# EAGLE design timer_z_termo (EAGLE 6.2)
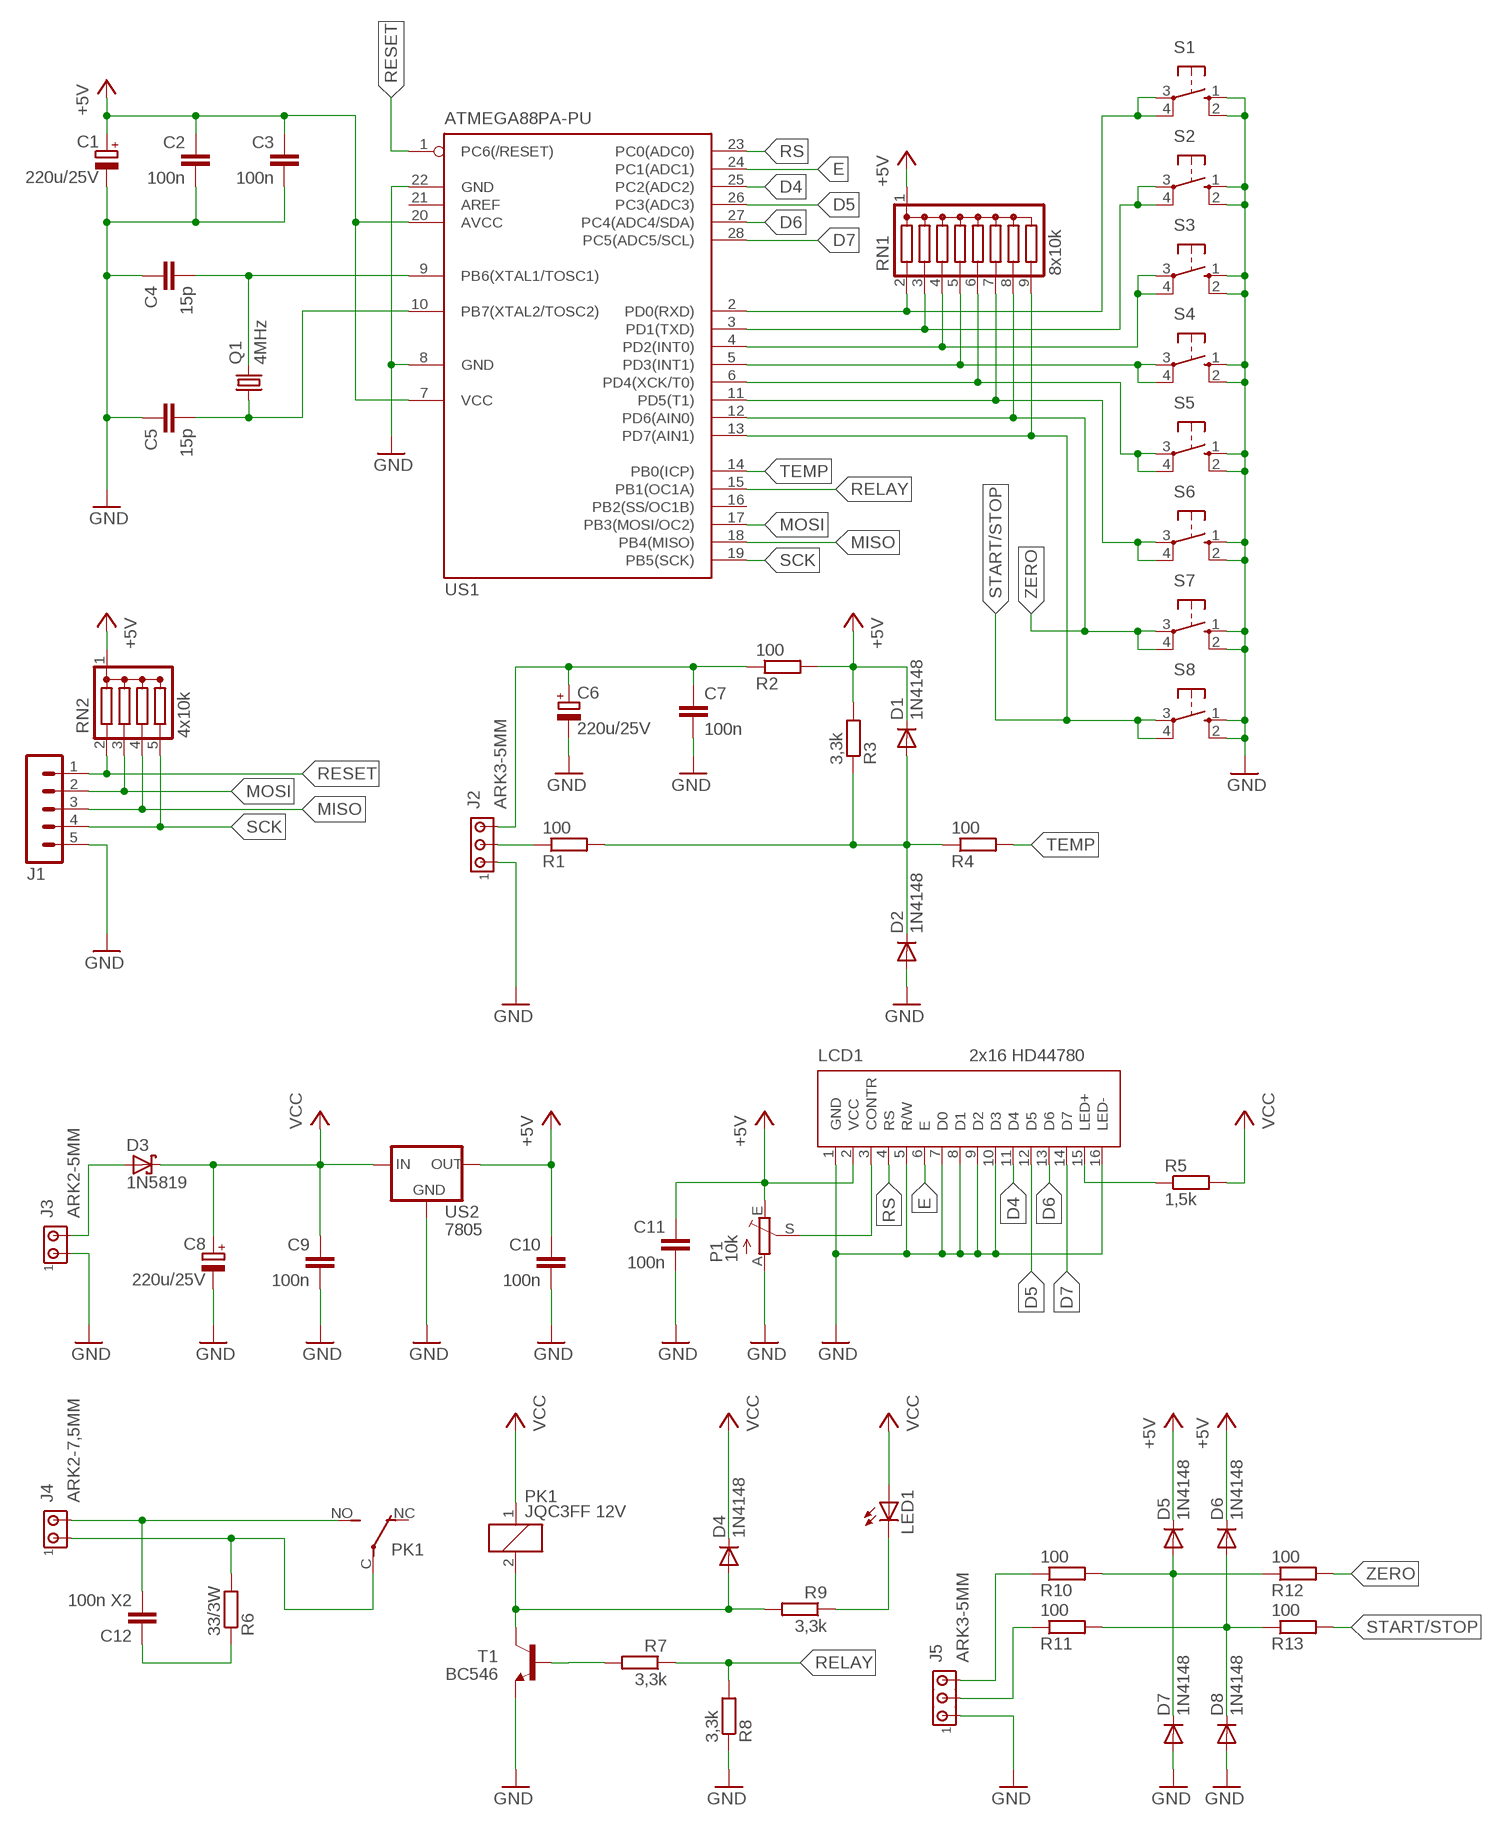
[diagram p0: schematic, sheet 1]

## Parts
C1  220u/25V  CPOL-EUE2.5-7  [E2,5-7]
C2  100n  C-EU050-025X075  [C050-025X075]
C3  100n  C-EU050-025X075  [C050-025X075]
C4  15p  C-EU050-025X075  [C050-025X075]
C5  15p  C-EU050-025X075  [C050-025X075]
C6  220u/25V  CPOL-EUE2.5-7  [E2,5-7]
C7  100n  C-EU050-025X075  [C050-025X075]
C8  220u/25V  CPOL-EUE2.5-7  [E2,5-7]
C9  100n  C-EU050-025X075  [C050-025X075]
C10  100n  C-EU050-025X075  [C050-025X075]
C11  100n  C-EU050-025X075  [C050-025X075]
C12  100n X2  C-EU102_152-062X184  [C102_152-062X184]
D1  1N4148  BAT81  [DO34-7]
D2  1N4148  BAT81  [DO34-7]
D3  1N5819  SCHOTTKY-DIODEF126Z12  [F126Z12]
D4  1N4148  BAT81  [DO34-7]
D5  1N4148  BAT81  [DO34-7]
D6  1N4148  BAT81  [DO34-7]
D7  1N4148  BAT81  [DO34-7]
D8  1N4148  BAT81  [DO34-7]
J1  MA05-1  [MA05-1]
J2  ARK3-5MM  [3PIN-5MM]
J3  ARK2-5MM  [2PIN-5MM]
J4  ARK2-7,5MM  [2PIN-7,5MM]
J5  ARK3-5MM  [3PIN-5MM]
LCD1  2x16 HD44780  LCD_2X16-NAD-ELEMENTAMI  [LCD_HD44780_2X16_NAD-ELEMENTAMI]
LED1  LED5MM  [LED5MM]
P1  10k  TRIM_EU-CA6V  [CA6V]
PK1  JQC3FF 12V  PK_POJED-JQC-3FG  [PK_POJED_JQC-3FG]
Q1  4MHz  CRYSTALHC49U-V  [HC49U-V]
R1  100  R-EU_0207/7  [0207/7]
R2  100  R-EU_0207/7  [0207/7]
R3  3,3k  R-EU_0207/7  [0207/7]
R4  100  R-EU_0207/7  [0207/7]
R5  1,5k  R-EU_0207/7  [0207/7]
R6  33/3W  R-EU_0617/17  [0617/17]
R7  3,3k  R-EU_0207/7  [0207/7]
R8  3,3k  R-EU_0207/7  [0207/7]
R9  3,3k  R-EU_0207/7  [0207/7]
R10  100  R-EU_0207/7  [0207/7]
R11  100  R-EU_0207/7  [0207/7]
R12  100  R-EU_0207/7  [0207/7]
R13  100  R-EU_0207/7  [0207/7]
RN1  8x10k  DRAB_REZ_1X8-SIL9  [RN-9]
RN2  4x10k  DRAB_REZ_1X4  [RN-5]
S1  10-XX  [B3F-10XX]
S2  10-XX  [B3F-10XX]
S3  10-XX  [B3F-10XX]
S4  10-XX  [B3F-10XX]
S5  10-XX  [B3F-10XX]
S6  10-XX  [B3F-10XX]
S7  10-XX  [B3F-10XX]
S8  10-XX  [B3F-10XX]
T1  BC546  BC546A  [TO92-EBC]
US1  ATMEGA88PA-PU  MEGA8-P  [DIL28-3]
US2  7805  78XXL  [78XXL]

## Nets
+5V: C1.+ C2.1 C3.1 C10.1 C11.1 D1.C D5.C D6.C LCD1.2(VCC) P1.E R2.2 R3.2 RN1.1(C) RN2.1(C) US1.7(VCC) US1.20(AVCC) US2.OUT
D4: LCD1.11(D4) US1.25(PC2(ADC2))
D5: LCD1.12(D5) US1.26(PC3(ADC3))
D6: LCD1.13(D6) US1.27(PC4(ADC4/SDA))
D7: LCD1.14(D7) US1.28(PC5(ADC5/SCL))
E: LCD1.6(E) US1.24(PC1(ADC1))
GND: C1.- C2.2 C3.2 C4.1 C5.1 C6.- C7.2 C8.- C9.2 C10.2 C11.2 D2.A D7.A D8.A J1.5 J2.P$1 J3.P$1 J5.P$1 LCD1.1(GND) LCD1.5(R/W) LCD1.7(D0) LCD1.8(D1) LCD1.9(D2) LCD1.10(D3) LCD1.16(LED-) P1.A R8.1 S1.1(S) S1.2(S1) S2.1(S) S2.2(S1) S3.1(S) S3.2(S1) S4.1(S) S4.2(S1) S5.1(S) S5.2(S1) S6.1(S) S6.2(S1) S7.1(S) S7.2(S1) S8.1(S) S8.2(S1) T1.E US1.8(GND) US1.22(GND) US2.GND
MISO: J1.3 RN2.4 US1.18(PB4(MISO))
MOSI: J1.2 RN2.3 US1.17(PB3(MOSI/OC2))
N$1: LCD1.3(CONTR) P1.S
N$2: C12.2 J4.P2 PK1.NO
N$3: C5.2 Q1.1 US1.10(PB7(XTAL2/TOSC2))
N$4: C4.2 Q1.2 US1.9(PB6(XTAL1/TOSC1))
N$5: RN1.2 S1.3(P) S1.4(P1) US1.2(PD0(RXD))
N$6: LCD1.15(LED+) R5.1
N$7: R7.2 T1.B
N$8: D3.A J3.P$2
N$9: D4.A PK1.2 R9.2 T1.C
N$10: RN1.3 S2.3(P) S2.4(P1) US1.3(PD1(TXD))
N$11: J4.P1 PK1.C(COM) R6.2
N$12: C12.1 R6.1
N$13: RN1.4 S3.3(P) S3.4(P1) US1.4(PD2(INT0))
N$14: RN1.5 S4.3(P) S4.4(P1) US1.5(PD3(INT1))
N$15: RN1.6 S5.3(P) S5.4(P1) US1.6(PD4(XCK/T0))
N$16: RN1.7 S6.3(P) S6.4(P1) US1.11(PD5(T1))
N$19: C6.+ C7.1 J2.P$3 R2.1
N$20: J2.P$2 R1.1
N$21: D1.A D2.C R1.2 R3.1 R4.1
N$22: LED1.K(C) R9.1
N$23: D5.A D7.C R10.2 R12.1
N$24: D6.A D8.C R11.2 R13.1
N$25: J5.P$2 R11.1
N$26: J5.P$3 R10.1
RELAY: R7.1 R8.2 US1.15(PB1(OC1A))
RESET: J1.1 RN2.2 US1.1(PC6(/RESET))
RS: LCD1.4(RS) US1.23(PC0(ADC0))
SCK: J1.4 RN2.5 US1.19(PB5(SCK))
START/STOP: R13.2 RN1.9 S8.3(P) S8.4(P1) US1.13(PD7(AIN1))
TEMP: R4.2 US1.14(PB0(ICP))
VCC: C8.+ C9.1 D3.C D4.C LED1.A PK1.1 R5.2 US2.IN
ZERO: R12.2 RN1.8 S7.3(P) S7.4(P1) US1.12(PD6(AIN0))
Unconnected: PK1.NC US1.16(PB2(SS/OC1B)) US1.21(AREF)

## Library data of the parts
C1 C6 C8 = rcl:CPOL-EU: POLARIZED CAPACITOR, European symbol
C2-C5 C7 C9-C12 = rcl:C-EU: CAPACITOR, European symbol
D1 D2 D4-D8 = diode:BAT81: DIODE
D3 = diode:SCHOTTKY-DIODE: Schottky Diode
J1 = zlacza_futrzak:MA05-1: PIN HEADER; OC_FARNELL: unknown; OC_NEWARK: unknown
J2 J5 = zlacza_futrzak:ARK3: ARK 3 Raster 5mm i 3,5mm
J3 J4 = zlacza_futrzak:ARK2: ARK 2
LCD1 = inne_futrzak:LCD_2X16
LED1 = led:LED: LED
P1 = pot:TRIM_EU-: POTENTIOMETER
PK1 = inne_futrzak:PK_POJED
Q1 = crystal:CRYSTAL: CRYSTAL; OC_FARNELL: 1666969; OC_NEWARK: unknown
R1-R13 = rcl:R-EU_: RESISTOR, European symbol
RN1 = inne_futrzak:DRAB_REZ_1X8
RN2 = inne_futrzak:DRAB_REZ_1X4
S1-S8 = switch-omron:10-XX: OMRON SWITCH; MPN: B3F-1000; OC_FARNELL: 176432; OC_NEWARK: 36M3542
T1 = transistor-npn:BC546*: NPN Transistor
US1 = atmel:MEGA8-P: MICROCONTROLLER 8 Kbytes FLASH, 1 kbytes SRAM, 512 bytes EEPROM, USART, 4-channel 10 bit ADC, 2-channel 8 bit ADC Pin compatible with Atmega48, ATMega88, ATMega168 Source: avr.lbr; OC_FARNELL: unknown; OC_NEWARK: unknown
US2 = v-reg:78XXL: VOLTAGE REGULATOR

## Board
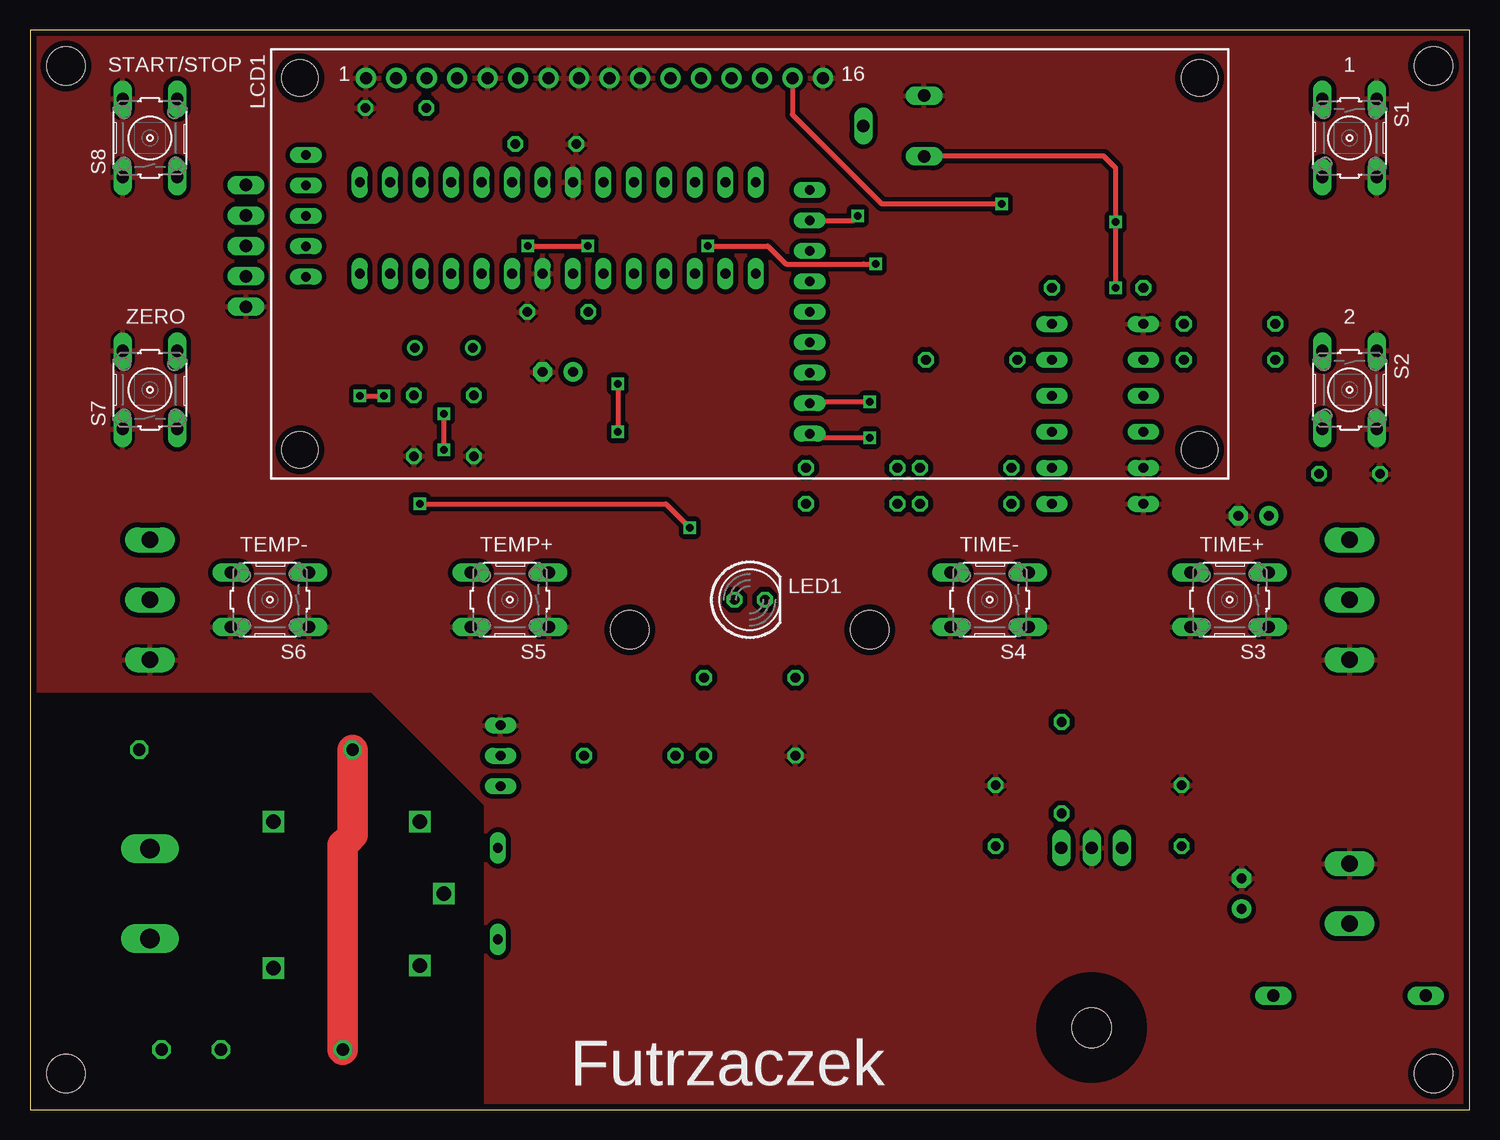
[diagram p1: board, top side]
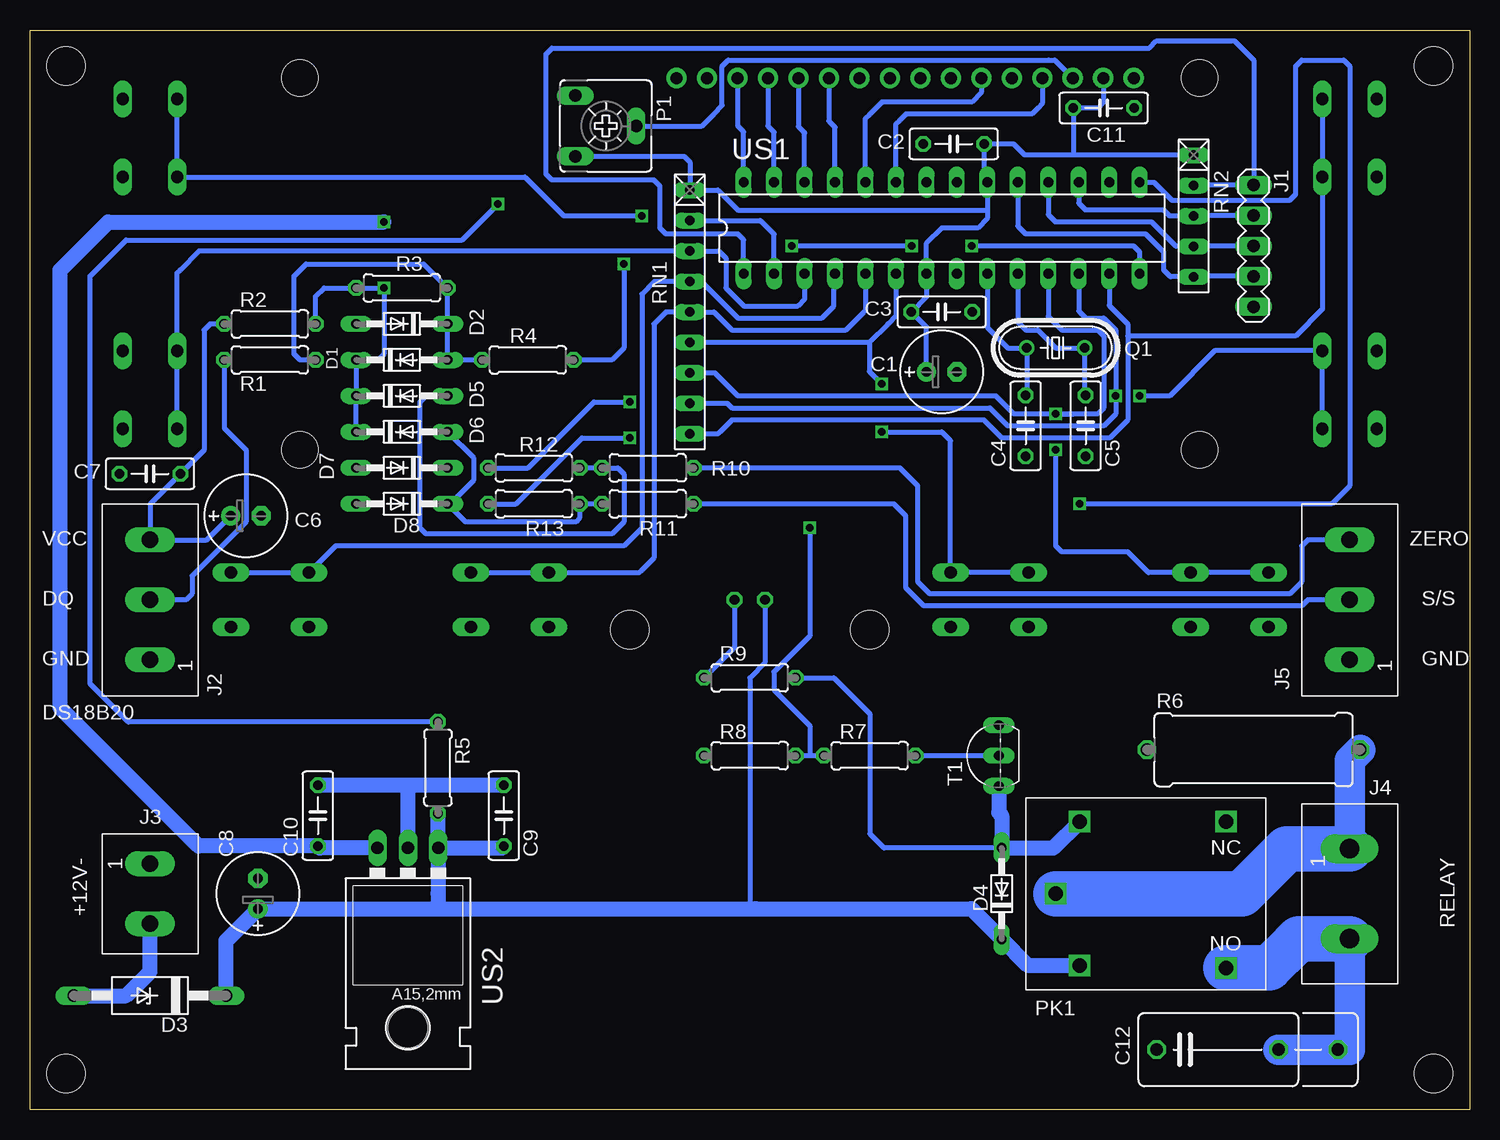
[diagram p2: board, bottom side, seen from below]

Size 120 x 90 mm. Coordinates in mm from the lower left corner, seen from the top.
Outline: 0,0 120,0 120,90 0,90 0,0
Copper layers (1*16): Top 0.035mm / dielectric 1.5mm / Bottom 0.035mm
Design rules: minimum track width 10mil, minimum drill 23mil, track to track 8mil, track to pad 8mil, pad to pad 8mil, via to via 8mil, smd to smd 8mil, copper to edge 20mil, drill to drill 8mil, minimum pad ring 10mil, minimum via ring 8mil, stop-mask expansion 4mil, vias tented up to drill 0mil, thermal gap 10mil
Holes 3.2 mm at 3,87 117,87 50,40 70,40 3,3 117,3

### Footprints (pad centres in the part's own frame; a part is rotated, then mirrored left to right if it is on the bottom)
E2,5-7 = drill 0.813 pad 1.6: + -1.27,0 | drill 0.813 pad 1.6 octagon: - 1.27,0
C050-025X075 = drill 0.813 octagon: 1 -2.54,0; 2 2.54,0
C102_152-062X184 = drill 1.016 octagon: 1 -5.08,0; 2 5.08,0; 3 10.033,0
DO34-7 = drill 0.813 long: A 3.81,0; C -3.81,0
F126Z12 = drill 1.016 long: A 6.35,0; C -6.35,0
MA05-1 = drill 1.016 long: 1 -5.08,0; 2 -2.54,0; 3 0,0; 4 2.54,0; 5 5.08,0
3PIN-5MM = drill 1.4 long: P$1 -5,0; P$2 0,0; P$3 5,0
2PIN-5MM = drill 1.4 long: P$1 -2.5,0; P$2 2.5,0
2PIN-7,5MM = drill 1.6 long: P1 -3.75,0; P2 3.75,0
LCD_HD44780_2X16_NAD-ELEMENTAMI = drill 1 pad 1.676: 1 -32,15.5; 2 -29.46,15.5; 3 -26.92,15.5; 4 -24.38,15.5; 5 -21.84,15.5; 6 -19.3,15.5; 7 -16.76,15.5; 8 -14.22,15.5; 9 -11.68,15.5; 10 -9.14,15.5; 11 -6.6,15.5; 12 -4.06,15.5; 13 -1.52,15.5; 14 1.02,15.5; 15 3.56,15.5; 16 6.1,15.5 | hole 3: -37.5,-15.5; 37.5,-15.5; -37.5,15.5; 37.5,15.5
LED5MM = drill 0.813 octagon: A -1.27,0; K 1.27,0
CA6V = drill 1.016 long: A -2.54,-2.54; E 2.54,-2.54; S 0,2.54
PK_POJED_JQC-3FG = drill 1.2 square: 1 5.5,6; 2 5.5,-6; C 7.5,0; NC -6.7,-6; NO -6.7,6.2
HC49U-V = drill 0.813: 1 -2.413,0; 2 2.413,0
0207/7 = drill 0.813 octagon: 1 -3.81,0; 2 3.81,0
0617/17 = drill 1.016 octagon: 1 -8.89,0; 2 8.89,0
RN-9 = drill 0.813 long: 1 -10.16,0; 2 -7.62,0; 3 -5.08,0; 4 -2.54,0; 5 0,0; 6 2.54,0; 7 5.08,0; 8 7.62,0; 9 10.16,0
RN-5 = drill 0.813 long: 1 -5.08,0; 2 -2.54,0; 3 0,0; 4 2.54,0; 5 5.08,0
B3F-10XX = drill 1.016 long: 1 -3.251,2.261; 2 3.251,2.261; 3 -3.251,-2.261; 4 3.251,-2.261
TO92-EBC = drill 0.813 long: B 0,-1.27; C -2.54,-1.27; E 2.54,-1.27
DIL28-3 = drill 0.813 long: 1 -16.51,-3.81; 2 -13.97,-3.81; 3 -11.43,-3.81; 4 -8.89,-3.81; 5 -6.35,-3.81; 6 -3.81,-3.81; 7 -1.27,-3.81; 8 1.27,-3.81; 9 3.81,-3.81; 10 6.35,-3.81; 11 8.89,-3.81; 12 11.43,-3.81; 13 13.97,-3.81; 14 16.51,-3.81; 15 16.51,3.81; 16 13.97,3.81; 17 11.43,3.81; 18 8.89,3.81; 19 6.35,3.81; 20 3.81,3.81; 21 1.27,3.81; 22 -1.27,3.81; 23 -3.81,3.81; 24 -6.35,3.81; 25 -8.89,3.81; 26 -11.43,3.81; 27 -13.97,3.81; 28 -16.51,3.81
78XXL = drill 1.016 long: GND 0,-3.81; IN -2.54,-3.81; OUT 2.54,-3.81 | hole 3.302: 0,11.176

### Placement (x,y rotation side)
C1  44,61.5 0 bottom
C2  43,80.5 180 bottom
C3  44,66.5 0 bottom
C4  37,57 90 bottom
C5  32,57 90 bottom
C6  102,49.5 0 bottom
C7  110,53 180 bottom
C8  101,18 90 bottom
C9  80.5,24.5 90 bottom
C10  96,24.5 90 bottom
C11  30.5,83.5 0 bottom
C12  21,5 0 bottom
D1  89,62.5 0 bottom
D2  89,65.5 180 bottom
D3  110,9.5 180 bottom
D4  39,18 90 bottom
D5  89,59.5 0 bottom
D6  89,56.5 0 bottom
D7  89,53.5 180 bottom
D8  89,50.5 180 bottom
J1  18,72 270 bottom
J2  110,42.5 90 bottom
J3  110,18 270 bottom
J4  10,18 270 bottom
J5  10,42.5 90 bottom
LCD1  60,70.5 0 top
LED1  60,42.5 0 top
P1  72,82 270 bottom
PK1  27,18 180 bottom
Q1  34.5,63.5 180 bottom
R1  100,62.5 0 bottom
R2  100,65.5 0 bottom
R3  89,68.5 180 bottom
R4  78.5,62.5 0 bottom
R5  86,28.5 270 bottom
R6  18,30 0 bottom
R7  50,29.5 0 bottom
R8  60,29.5 0 bottom
R9  60,36 0 bottom
R10  68.5,53.5 180 bottom
R11  68.5,50.5 180 bottom
R12  78,53.5 180 bottom
R13  78,50.5 180 bottom
RN1  65,66.5 270 bottom
RN2  23,74.5 270 bottom
S1  110,81 270 top
S2  110,60 270 top
S3  100,42.5 180 top
S4  80,42.5 180 top
S5  40,42.5 180 top
S6  20,42.5 180 top
S7  10,60 90 top
S8  10,81 90 top
T1  40.5,29.5 90 bottom
US1  44,73.5 0 bottom
US2  88.5,18 180 bottom

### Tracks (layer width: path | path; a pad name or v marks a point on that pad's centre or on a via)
+5V  (via drill 0.6)
  Top 0.406: v90.5,68.5 v90.5,74 90.5,78.5 89.5,79.5 74.58,79.5 P1.E
  Bottom 0.406: 40.19,75 US1.20 40.46,77.58 C2.1 38,80.5 37.08,79.58 33,79.58 | 40.19,75 40.19,74.31 41,73.5 44,73.5 45.27,72.23 US1.7 45.27,67.77 C3.1 45.27,65.23 C1.+ | RN2.1 33,79.58 | 33,79.58 33.04,79.62 C11.1 31,83.5 30.54,83.96 LCD1.2 | 40.19,75 61,75 62.66,76.66 RN1.1 65,79 65.46,79.46 P1.E | D6.C D5.C D1.C 91,62.5 90.5,63 v90.5,68.5 R3.2 95.5,68.5 96.19,67.81 R2.2
  Bottom 1.27: US2.OUT 95.85,21.81 C10.1 105.96,21.96 117.5,33.5 117.5,70 113.5,74 v90.5,74
D4
  Bottom 0.406: US1.25 52.89,81.89 53,82 53.4,82.4 LCD1.11
D5
  Bottom 0.406: US1.26 55.43,81.43 55.94,81.94 LCD1.12
D6
  Bottom 0.406: US1.27 57.97,81.47 58.48,81.98 LCD1.13
D7
  Bottom 0.406: US1.28 60.51,81.51 61,82 61.02,82.02 LCD1.14
E
  Bottom 0.406: LCD1.6 40.7,84.8 41.5,84 49,84 50,83 50.35,82.65 US1.24
GND
  Bottom 1.27: C9.2 88.5,27.04 | 88.5,27.04 C10.2 | US2.GND 88.5,27.04
  pour Top (isolate 0.406): 0,35 28.5,35 38,25.5 38,0 120,0 120,90 0,90
MISO
  Bottom 0.406: J1.3 22.96,72 RN2.4 24.46,71.96 26.5,74 34.5,74 35.11,74.61 US1.18
MOSI
  Bottom 0.406: J1.2 22.96,74.54 RN2.3 25,74.5 25.5,75 32,75 32.57,75.57 US1.17
N$1
  Bottom 0.406: P1.S 64,82 63,83 62.3,83.7 62.3,87 61.8,87.5 35.08,87.5 34.58,87.5 LCD1.3
N$2
  Bottom 2.54: J4.P2 10,5 C12.2
  Bottom 3.81: PK1.NO 16.7,11.8 14.75,13.75 | 14.75,13.75 14.5,14 | J4.P2 14.25,14.25 14.75,13.75
N$3
  Bottom 0.406: US1.10 37.65,65.65 37,65 36,65 34.5,63.5 Q1.1 32.09,59.63 C5.2
N$4
  Bottom 0.406: US1.9 40.19,65.19 38.5,63.5 Q1.2 36.91,59.63 C4.2
N$5  (via drill 0.6)
  Top 0.406: RN1.2 68.62,74.12 v69,74.5
  Bottom 0.406: RN1.2 59.12,74.12 58,73 57.97,72.97 US1.2 | v69,74.5 75.5,74.5 78.5,77.5 78.75,77.75 S1.4 S1.3
N$6  (via drill 0.6)
  Top 0.406: v81,75.5 71,75.5 66,80.5 63.56,82.94 LCD1.15
  Bottom 0.406: R5.1 111.81,32.31 113.5,34 115,35.5 115,69.5 112,72.5 84,72.5 v81,75.5
N$7
  Bottom 0.406: T1.B R7.2
N$8
  Bottom 1.27: D3.A 112,9.5 110,11.5 J3.P$2
N$9
  Bottom 0.406: R9.2 53,36 50,33 50,23 49,22 48.81,21.81 D4.A
  Bottom 1.27: T1.C 39.23,24.73 39,24.5 D4.A 34.69,21.81 PK1.2
N$10
  Bottom 0.406: US1.3 55.43,67.57 56,67 60.5,67 62,68.5 62,71 62.58,71.58 RN1.3 105.92,71.58 107.5,70 107.74,69.76 S2.3 S2.4
N$11
  Bottom 2.54: J4.P1 10,29.11 R6.2
  Bottom 3.81: PK1.C 19,18 15.5,21.5 15.25,21.75 J4.P1
N$12
  Top 2.54: C12.1 26.08,22.08 26.5,22.5 26.89,22.89 R6.1
N$13
  Bottom 0.406: US1.4 53,69.58 53,67 54,66 61,66 63,68 64.04,69.04 RN1.4 67.96,69.04 69,68 69,48.5 70.5,47 94.51,47 S3.4 S3.3
N$14
  Bottom 0.406: US1.5 50.35,66.65 50.5,66.5 52,65 61.5,65 63,66.5 RN1.5 67,66.5 68,65.5 68,46 69,45 69.24,44.76 S4.4 S4.3
N$15  (via drill 0.6)
  Top 0.406: v49,60.5 v49,56.5
  Bottom 0.406: RN1.6 50.04,63.96 | 50.04,63.96 48.5,65.5 47.81,66.19 US1.6 | S5.4 S5.3 43.25,55.75 43.5,56 44,56.5 v49,56.5 | 50.04,63.96 50.04,61.54 v49,60.5
N$16  (via drill 0.6)
  Top 0.406: v34.5,55 v34.5,58
  Bottom 0.406: US1.11 35.11,66.11 34,65 31,65 30.5,64.5 30.5,58.5 31,58 33,58 | 33,58 v34.5,58 | v34.5,58 38,58 39.5,59.5 61,59.5 62.25,60.75 | 62.25,60.75 62.5,61 | RN1.7 62.92,61.42 62.25,60.75 | S6.4 S6.3 26.76,44.76 27.5,45.5 28.5,46.5 34,46.5 34.5,47 v34.5,55 | v34.5,58 33,58
N$19
  Bottom 0.406: C6.+ 105.27,47.5 J2.P$3 110,50.46 C7.1 105.5,54.96 105.5,65 105,65.5 R2.1
N$20
  Bottom 0.406: R1.1 103.81,56.81 102,55 102,49 106.5,44.5 106.5,43 107,42.5 J2.P$2
N$21
  Bottom 0.406: R4.1 D1.A D2.C R3.1 87.19,70.5 97,70.5 98,69.5 98,63 97.5,62.5 R1.2
N$22
  Bottom 0.406: LED1.K 61.27,38.54 R9.1
N$23
  Bottom 0.406: D7.C 87,53.5 87.5,53.5 | R12.1 R10.2 71,53.5 70.5,53 70.5,49 71.5,48 87,48 87.5,48.5 87.5,53 87.5,53.5 | 87.5,53.5 87.5,59 87,59.5 D5.A
N$24
  Bottom 0.406: R11.2 R13.1 74.19,49.31 74.5,49 83.69,49 D8.C 85,50.5 83,52.5 83,54.31 D6.A
N$25
  Bottom 0.406: J5.P$2 13.5,42.5 14,42 45.5,42 47,43.5 47,49.5 48,50.5 R11.1
N$26
  Bottom 0.406: J5.P$3 13.5,47.5 14,47 14,44 15,43 45,43 46,44 46,52 47.5,53.5 R10.1
RELAY  (via drill 0.6)
  Top 0.406: v32.5,50.5 53,50.5 v55,48.5
  Bottom 0.406: R7.1 55,29.5 | 55,29.5 R8.2 | US1.15 26.31,77.31 24.8,75.8 15,75.8 14.5,76.3 14.5,87 14,87.5 10.5,87.5 10,87 10,52 10.5,51.5 11.5,50.5 v32.5,50.5 | v55,48.5 55,39.5 58,36.5 58,35 55,32 55,29.5
RESET
  Bottom 0.406: RN2.2 22.96,77.08 J1.1 18,87.5 19,88.5 19.6,89.1 26.1,89.1 26.7,88.5 76.5,88.5 77,88 77,78 76.5,77.5 68,77.5 67.5,77 67.5,73.5 67,73 61,73 60.51,72.51 US1.1
RS
  Bottom 0.406: LCD1.4 35.62,83.88 36,83.5 36.5,83 47,83 47.5,82.5 47.81,82.19 US1.23
SCK
  Bottom 0.406: J1.4 22.96,69.46 RN2.5 23.92,69.42 24.92,69.42 25.5,70 25.5,71.5 26.5,72.5 27,73 37,73 37.5,73.5 37.65,73.65 US1.19
START/STOP  (via drill 0.6)
  Top 0.406: v70,56 65.34,56 RN1.9
  Bottom 0.406: US1.13 30.03,67.03 28.5,65.5 28.5,64.5 | 28.5,64.5 28.5,57.5 30,56 39,56 40.5,57.5 61.5,57.5 62,57 | 62,57 62.5,56.5 | RN1.9 62.66,56.34 62,57 | S8.4 S8.3 12.26,66.74 14.5,64.5 28.5,64.5 | R13.2 79.5,50.5 74,56 v70,56
TEMP  (via drill 0.6)
  Top 0.406: v41.5,72 v46.5,72 | v56.5,72 61.5,72 62.5,71 63,70.5 69.5,70.5 v70.5,70.5
  Bottom 0.406: US1.14 27.49,71.49 28,72 v41.5,72 | v46.5,72 v56.5,72 | v70.5,70.5 70.5,63.5 71.5,62.5 R4.2
VCC
  Bottom 0.406: LED1.A 58.73,37.27 60,36 60,17.23 59.5,16.73
  Bottom 1.27: D3.C 103.65,14.08 C8.+ 86,16.73 | US2.IN 85.96,18.04 86,18 86,16.73 | US2.IN 80.65,21.81 C9.1 | US2.IN 85.96,24.65 R5.2 | PK1.1 36.81,12 D4.C 41.54,16.73 59.5,16.73 86,16.73
ZERO  (via drill 0.6)
  Top 0.406: v27.5,59.5 v29.5,59.5 | v70,59 65.12,59 RN1.8
  Bottom 0.406: US1.12 32.57,66.57 32,66 30.5,66 29.5,65 29.5,60 | 29.5,60 v29.5,59.5 | v29.5,59.5 29.5,58 30.5,57 38.5,57 40,58.5 61.5,58.5 61.88,58.88 RN1.8 | S7.3 S7.4 21.25,63.25 25,59.5 v27.5,59.5 | v29.5,59.5 29.5,60 | R12.2 78.5,53.5 73,59 v70,59

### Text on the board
tPlace: START/STOP | 1 | ZERO | 2 | TEMP- | TEMP+ | TIME- | TIME+ | Futrzaczek
bPlace: ZERO | VCC | S/S | DQ | GND | GND | DS18B20 | RELAY | +12V-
